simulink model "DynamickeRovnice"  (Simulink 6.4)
settings: Solver=ode45  StartTime=0.0  StopTime=10  MaxStep=1e-2  RelTol=1e-3

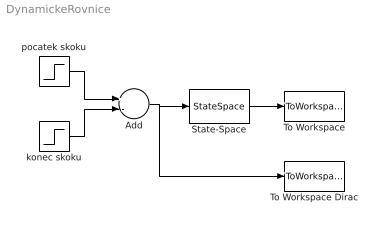
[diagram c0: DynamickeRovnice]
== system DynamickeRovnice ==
  Add : Sum  Inputs=+-  OutScaling=2^-10
  State-Space : StateSpace  A=[-1, 0; 0, -2]  B=[1; 1]  C=[6, -3]  D=[0]
  To Workspace : ToWorkspace  VariableName=y  SampleTime=-1  SaveFormat=Structure With Time
  To Workspace Dirac : ToWorkspace  VariableName=dirac  SampleTime=-1  SaveFormat=Structure With Time
  konec skoku : Step  Time=3  After=0.5  SampleTime=0
  pocatek skoku : Step  After=0.5  SampleTime=0
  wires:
  State-Space/1 -> To Workspace/1
  Add/1 -> State-Space/1, To Workspace Dirac/1
  pocatek skoku/1 -> Add/1
  konec skoku/1 -> Add/2
